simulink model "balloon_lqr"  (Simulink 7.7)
settings: Solver=ode45  StartTime=0.0  StopTime=50000  RelTol=1e-3
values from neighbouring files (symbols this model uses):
  C = V*rho_a*c_a    [balloon_init.m]
  f = f / 10    [balloon_init.m]
  g = 9.80665    [balloon_init.m]
  m = input('Inserire le prime due cifre (esclusi zeri) del proprio numero di matricola:\n\n')    [balloon_init.m]
  rho_a = 1.2928    [balloon_init.m]
  Ta = 20+273.15    (= 293.15)    [balloon_init.m]
  theta_t = theta_t/50    [balloon_init.m]
  V = V*m*2    [balloon_init.m]
  x1_0 = x1_d    [balloon_init.m]
  x2_0 = 100    [balloon_init.m]
  x2_d = 120    [balloon_init.m]
  x3_0 = 0    [balloon_init.m]
  x3_d = 0    [balloon_init.m]
undefined symbols (not defined in the file or in its folder): K
libraries: simulink x2

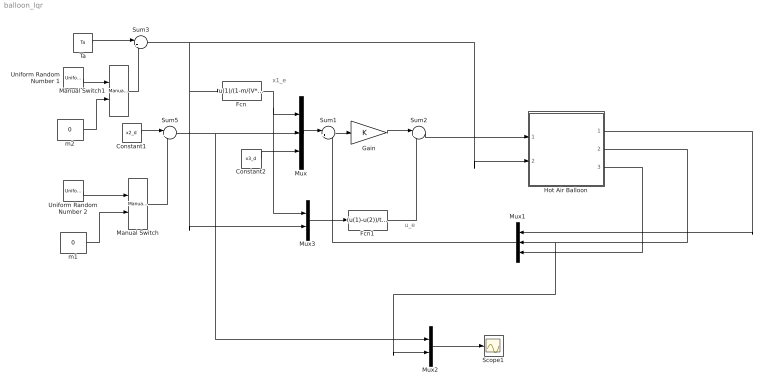
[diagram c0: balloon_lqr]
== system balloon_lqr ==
  note: x1_e
  note: u_e
  Constant1 : Constant  Value=x2_d
  Constant2 : Constant  Value=x3_d
  Fcn : Fcn  Expr=u(1)/(1-m/(V*rho_a))
  Fcn1 : Fcn  Expr=(u(1)-u(2))/theta_t
  Gain : Gain  Gain=K  Multiplication=Matrix(K*u)
  Hot Air Balloon : Subsystem  mask{V=V, m=m, C=C, theta_t=theta_t, f=f, g=g}
      mask prompts: V "Balloon's volume (V)"; m "Balloon's total mass (m)"; C "Thermal capacitance (C)"; theta_t "Thermal resistance (theta_t)"; f "Aerodynamic viscous friction (f)"; g "Gravitational acceleration (g)"
  Manual Switch : simulink/Signal Routing/Manual Switch  SystemSampleTime=-1  sw=1  action=0  varsize=off
  Manual Switch1 : simulink/Signal Routing/Manual Switch  SystemSampleTime=-1  sw=0  action=0  varsize=off
  Mux : Mux  Inputs=3
  Mux1 : Mux  Inputs=3
  Mux2 : Mux  Inputs=2
  Mux3 : Mux  Inputs=2
  Scope1 : Scope
  Sum1 : Sum  Inputs=|+-
  Sum2 : Sum  Inputs=|++
  Sum3 : Sum  Inputs=|++
  Sum5 : Sum  Inputs=|++
  Ta : Constant  Value=Ta
  Uniform Random Number 1 : UniformRandomNumber  SampleTime=200
  Uniform Random Number 2 : UniformRandomNumber  Minimum=-x2_d*0.1  Maximum=x2_d*0.1  Seed=1  SampleTime=1500
  m1 : Constant  Value=0
  m2 : Constant  Value=0
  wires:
  Constant2/1 -> Mux/3
  Mux/1 -> Sum1/1
  Sum1/1 -> Gain/1
  Gain/1 -> Sum2/1
  Fcn1/1 -> Sum2/2
  Mux1/1 -> Sum1/2
  Mux2/1 -> Scope1/1
  Sum2/1 -> Hot Air Balloon/1(u)
  Hot Air Balloon/3(x3) -> Mux1/3
  Hot Air Balloon/2(x2) -> Mux1/2, Mux2/2
  Hot Air Balloon/1(x1) -> Mux1/1
  Ta/1 -> Sum3/1
  Constant1/1 -> Sum5/1
  Sum5/1 -> Mux/2, Mux2/1
  Sum3/1 -> Fcn/1, Mux3/2, Hot Air Balloon/2(Ta)
  Fcn/1 -> Mux/1, Mux3/1
  Mux3/1 -> Fcn1/1
  Uniform Random Number 2/1 -> Manual Switch/1
  Manual Switch/1 -> Sum5/2
  m1/1 -> Manual Switch/2
  m2/1 -> Manual Switch1/2
  Manual Switch1/1 -> Sum3/2
  Uniform Random Number 1/1 -> Manual Switch1/1

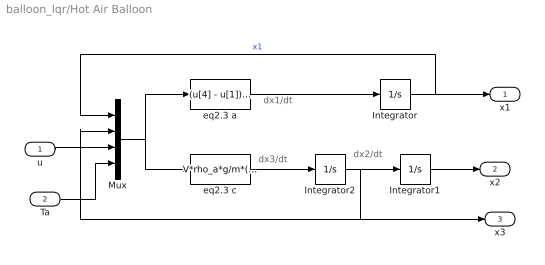
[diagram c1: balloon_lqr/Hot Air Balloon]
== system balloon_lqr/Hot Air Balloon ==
  note: dx2/dt
  note: dx3/dt
  note: dx1/dt
  u : Inport
  Ta : Inport  Port=2
  Integrator : Integrator  InitialCondition=x1_0
  Integrator1 : Integrator  InitialCondition=x2_0  LowerSaturationLimit=0
  Integrator2 : Integrator  InitialCondition=x3_0
  Mux : Mux
  eq2.3 a : Fcn  Expr=(u[4] - u[1])/(C*theta_t) + u[3]/C
  eq2.3 c : Fcn  Expr=V*rho_a*g/m*(1 - u[4]/u[1]) - f/m*u[2] - g
  x1 : Outport
  x2 : Outport  Port=2
  x3 : Outport  Port=3
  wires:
  Ta/1 -> Mux/4
  u/1 -> Mux/3
  Integrator1/1 -> x2/1
  Integrator2/1 -> Mux/2, x3/1, Integrator1/1
  Integrator/1 -> x1/1, Mux/1  "x1"
  Mux/1 -> eq2.3 c/1, eq2.3 a/1
  eq2.3 c/1 -> Integrator2/1
  eq2.3 a/1 -> Integrator/1
